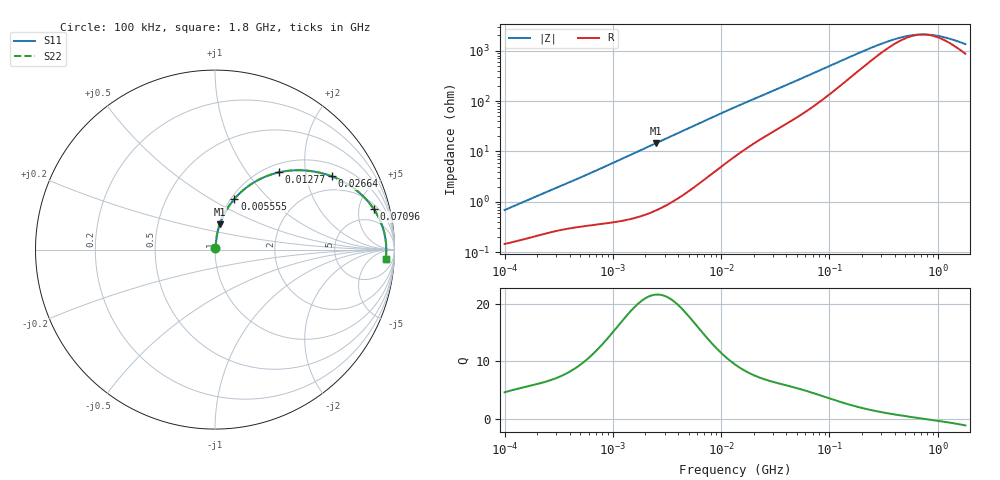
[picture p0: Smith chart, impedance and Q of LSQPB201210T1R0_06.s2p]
! LSQPB201210T1R0_06  S-PARAMETER MODEL  ( General Type )
! Model Generated by TAIYO YUDEN Corporation (http://www.ty-top.com)
! Version 1.0
! TAIYO YUDEN Control No. 120417NG38SB-FKC
! Copyright(c) 2012 TAIYO YUDEN CO.,LTD. All Rights Reserved.
! Product Description (link to TY-COMPAS)
! https://ds.yuden.co.jp/TYCOMPAS/or/detail?pn=LSQPB201210T1R0M06&u=M
! Products Name : Inductors
! Characteristics :
!  Inductance : 1.0 uH , SRF(min) : 400 MHz , DC Resistance(max) : 0.1404 Ohm
!  Rated Current : Saturation :1050 mA , Temp Rise : 1230 mA (40 degC)
!  Case Size : 2.0 x 1.25 / 0.079 x 0.049 [mm/inch] , Thickness : 1.0 / 0.04 [mm/inch]
!  (Conditions: Temperature = 25 degC , DC Bias Current/Voltage = 0A / 0V)
! External Node Assignments :
!  1  o---GGG---o  2
! GND o---------o GND
! Frequency Range : 0.1MHz  -  1800MHz  [ 402 STEP ]
# MHz S RI R 50
! Freq[MHz].  S11 Real  S11 Imag  S21 Real  S21 Imag  S12 Real  S12 Imag  S22 Real  S22 Imag
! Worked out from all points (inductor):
!   401 points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, 100 kHz to 1.8 GHz, reference 50 ohm
!   read as one part in series: L = 1.06 uH near 105 kHz
!   highest Q = 21.6 at 2.475 MHz (marker M1), where L = 932 nH
!   self-resonance near 727.3 MHz
!   S11 on the Smith chart (normalised r, x): 100 kHz: 1.00, +0.01; 5.555 MHz: 1.04, +0.65; 12.77 MHz: 1.15, +1.44; 26.64 MHz: 1.42, +2.83; 70.96 MHz: 2.57, +6.97; 1.8 GHz: 18, -21
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0.1  0.00151 0.00673  0.9985 -0.00673  0.9985 -0.00673  0.00151 0.00673
0.516129  0.0042 0.0309  0.9958 -0.0309  0.9958 -0.0309  0.0042 0.0309
1.216451  0.00924 0.0707  0.9908 -0.0707  0.9908 -0.0707  0.00924 0.0707
2.475151  0.0268 0.1401  0.9732 -0.1401  0.9732 -0.1401  0.0268 0.1401
2.66389  0.0304 0.1501  0.9696 -0.1501  0.9696 -0.1501  0.0304 0.1501
3.942096  0.06 0.2138  0.94 -0.2138  0.94 -0.2138  0.06 0.2138
5.554714  0.1081 0.2823  0.8919 -0.2823  0.8919 -0.2823  0.1081 0.2823
8.220015  0.2011 0.3645  0.7989 -0.3645  0.7989 -0.3645  0.2011 0.3645
12.77497  0.3573 0.4306  0.6427 -0.4306  0.6427 -0.4306  0.3573 0.4306
13.41641  0.3771 0.4346  0.6229 -0.4346  0.6229 -0.4346  0.3771 0.4346
18.44729  0.5085 0.4404  0.4915 -0.4404  0.4915 -0.4404  0.5085 0.4404
26.63823  0.6502 0.4081  0.3498 -0.4081  0.3498 -0.4081  0.6502 0.4081
42.42587  0.7901 0.3285  0.2099 -0.3285  0.2099 -0.3285  0.7901 0.3285
69.24595  0.8805 0.232  0.1195 -0.232  0.1195 -0.232  0.8805 0.232
70.9631  0.8836 0.2274  0.1164 -0.2274  0.1164 -0.2274  0.8836 0.2274
151.6408  0.9382 0.1118  0.0618 -0.1118  0.0618 -0.1118  0.9382 0.1118
357.3983  0.9524 0.0384  0.0476 -0.0384  0.0476 -0.0384  0.9524 0.0384
542.0029  0.9541 0.0149  0.0459 -0.0149  0.0459 -0.0149  0.9541 0.0149
659.3364  0.9544 0.00491  0.0456 -0.00491  0.0456 -0.00491  0.9544 0.00491
782.6622  0.9544 -0.00367  0.0456 0.00367  0.0456 0.00367  0.9544 -0.00367
1130.179  0.9539 -0.0227  0.0461 0.0227  0.0461 0.0227  0.9539 -0.0227
1800  0.9517 -0.0516  0.0483 0.0516  0.0483 0.0516  0.9517 -0.0516
